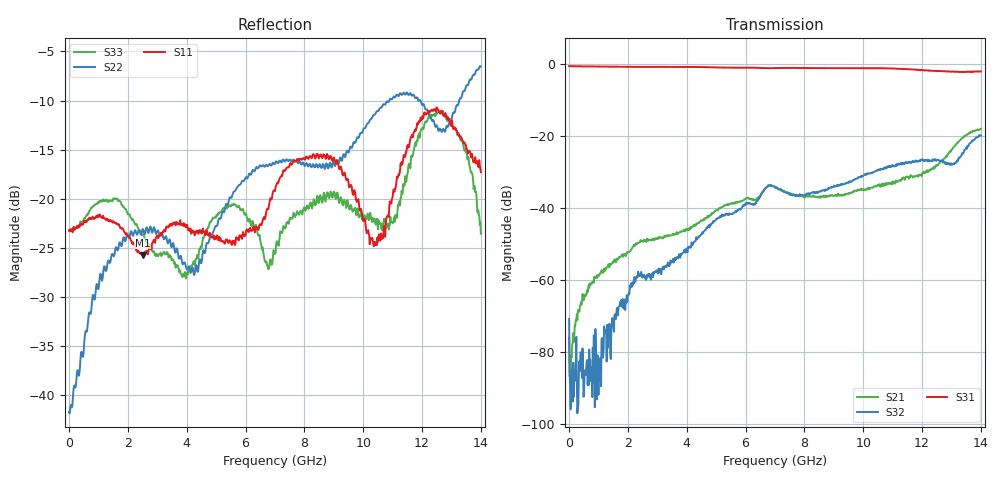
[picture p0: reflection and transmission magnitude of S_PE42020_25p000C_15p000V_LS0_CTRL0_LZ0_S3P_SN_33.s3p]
! Device ID: PE42020
! File Path: z:\PE42020\sparam_retest1\25p000C\3p000\LS_CTRL0_LZ0\PE42020_25p000C_3p000V_3p000V_0p000V_LS_CTRL0_LZ0_S3P_SN_33__2_3.s3p
! Serial: 33
! Lot:
! Temp: 25.000C
! VDD: 15.000
! VSS: -15.000
! Control_Hi: 3.000
! Control_Lo: 0.000
! Logic State: LS_CTRL0_LZ0
! Port 1: RFC
! Port 3: RF2
! Port 4:
! ThroughPath:1-4
! IDD: -0.0020740302
! ISS: 0
! Comment:
#  Hz  S  RI  R  50
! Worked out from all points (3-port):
!   801 points, 300 kHz to 14 GHz, reference 50 ohm
!   strongest paths, dB at 300 kHz, 3.5 GHz, 7 GHz, 10.5 GHz, 14 GHz:
!     S31: -0.6, -0.8, -1.1, -1.1, -2.1
!     S32: -70.7, -54.7, -34.1, -29.5, -19.9
!     S21: -75.9, -47.4, -34.1, -33.5, -18.0
!   lowest |S11| = -25.7 dB at 2.503 GHz (marker M1), VSWR 1.11, Z = 54.2 - j3.41 ohm
!   |S11| at or under -10 dB: start of sweep to end of sweep
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300000  0.0687 0.00408  -0.000798 -2.99e-05  0.9342 2.44e-05
        -6.27e-05 0.000148  0.00814 -0.00104  7.51e-05 2.78e-05
        0.9342 0.000691  0.000282 -7.62e-05  0.0689 0.00366
8.78e7  0.0695 -0.00771  1.16e-05 6.44e-05  0.9322 -0.0241
        -2.09e-07 8.48e-05  0.00841 -0.00205  4.67e-06 4.43e-05
        0.9328 -0.0235  -1.71e-05 -3.73e-05  0.069 -0.00661
1.0153e9  0.0532 -0.0612  9.8e-06 0.00117  0.8927 -0.2391
          -1.05e-05 0.00119  0.0259 -0.0251  -6.71e-05 1.79e-05
          0.8925 -0.2396  -3.74e-05 -6.45e-05  0.0666 -0.0684
2.5028e9  0.041 -0.0314  0.000182 0.00337  0.7342 -0.5436
          0.00025 0.00349  0.0658 -0.0242  -0.00106 0.000415
          0.7336 -0.5424  -0.000979 0.000534  0.049 -0.0433
4.3053e9  0.0373 -0.057  -0.000481 0.00575  0.4129 -0.8101
          -0.00048 0.00571  0.0248 -0.0383  -0.00324 0.00137
          0.4161 -0.8102  -0.00325 0.00134  0.0081 -0.0486
7.0003e9  0.0508 -0.0969  0.0132 0.0149  -0.1704 -0.864
          0.013 0.0148  0.0144 -0.1499  0.00652 0.0183
          -0.169 -0.8623  0.00633 0.0186  0.0351 -0.0394
8.9428e9  0.0827 -0.1342  0.0109 0.00979  -0.5663 -0.6708
          0.0109 0.0107  -0.0837 -0.1206  0.0126 0.0147
          -0.5595 -0.6745  0.0128 0.0151  0.0502 -0.0886
1.03953e10  0.00341 -0.0603  0.0129 0.0157  -0.7797 -0.4023
            0.0132 0.0151  -0.2634 -0.0532  0.0287 0.0154
            -0.7753 -0.4083  0.0286 0.0152  -0.0503 -0.0563
1.26003e10  -0.0837 -0.2641  0.0182 0.0374  -0.7934 0.0885
            0.0186 0.0378  -0.115 0.1959  0.043 -0.0152
            -0.7953 0.0816  0.0433 -0.0146  0.0312 -0.2758
1.40003e10  0.12 -0.0653  0.1178 0.0425  -0.7189 0.3209
            0.1187 0.0435  0.3009 0.3625  0.0937 -0.0418
            -0.7247 0.3114  0.0942 -0.0383  0.0286 -0.0598
